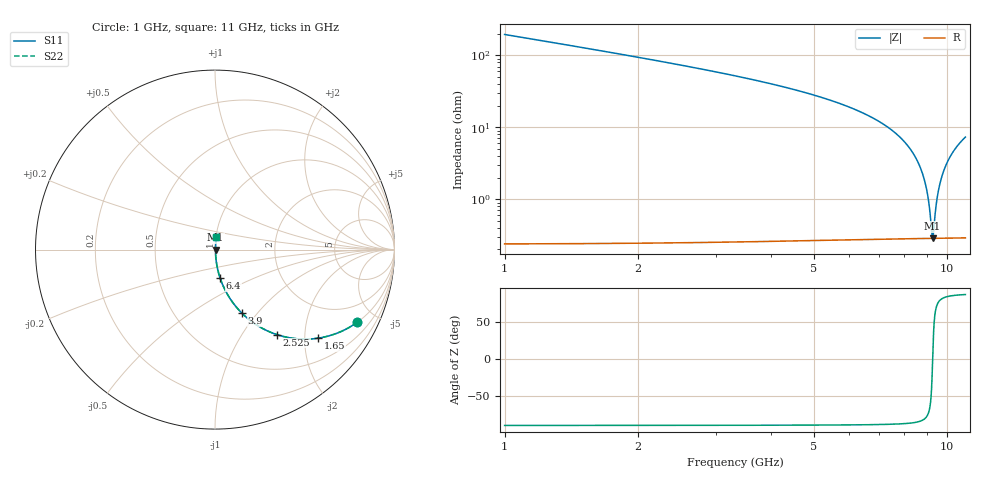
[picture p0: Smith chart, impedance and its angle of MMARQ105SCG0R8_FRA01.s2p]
! MMARQ105SCG0R8_FRA01  S-PARAMETER MODEL  ( General Type )
! Model Generated by TAIYO YUDEN Corporation (http://www.ty-top.com)
! Version 1.0
! TAIYO YUDEN Control No. 200326
! Copyright(c) 2020 TAIYO YUDEN CO.,LTD. All Rights Reserved.
! Product Description (link to TY-COMPAS)
! https://ds.yuden.co.jp/TYCOMPAS/or/detail?pn=MMARQ105SCG0R8BFRA01&u=M
! Products Name : Multilayer Ceramic Capacitors
! Characteristics :
!  Capacitance : 0.8 pF , Rated Voltage : 250V , TCC : CG / C0G
!  Case Size : 1.0 x 0.5 / 0.039 x 0.02 [mm/inch] , Thickness : 0.5 / 0.02 [mm/inch]
!  (Conditions: Temperature = 25 degC , DC Bias Current/Voltage = 0A / 0V)
! External Node Assignments :
!  1  o---| |---o  2
! GND o---------o GND
! Frequency Range : 1GHz  -  11GHz  [ 401 STEP ]
# MHz S RI R 50
! Freq[MHz].  S11 Real  S11 Imag  S21 Real  S21 Imag  S12 Real  S12 Imag  S22 Real  S22 Imag
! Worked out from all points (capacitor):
!   401 points, 1 GHz to 11 GHz, reference 50 ohm
!   read as one part in series: C = 802 fF near 1.05 GHz
!   lowest |Z| = 286 mohm at 9.275 GHz (marker M1)
!   series resonance near 9.276 GHz, so ESL is about 370 pH
!   S11 on the Smith chart (normalised r, x): 1 GHz: 1.00, -3.92; 1.65 GHz: 1.00, -2.33; 2.525 GHz: 1.00, -1.45; 3.9 GHz: 1.01, -0.84; 6.4 GHz: 1.01, -0.32; 11 GHz: 1.01, +0.15
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1000  0.7934 -0.4043  0.2066 0.4043  0.2066 0.4043  0.7934 -0.4043
1650  0.5754 -0.4932  0.4246 0.4932  0.4246 0.4932  0.5754 -0.4932
2525  0.3466 -0.4742  0.6534 0.4742  0.6534 0.4742  0.3466 -0.4742
2675  0.3168 -0.4634  0.6832 0.4634  0.6832 0.4634  0.3168 -0.4634
3900  0.1507 -0.3547  0.8493 0.3547  0.8493 0.3547  0.1507 -0.3547
4350  0.1141 -0.3143  0.8859 0.3143  0.8859 0.3143  0.1141 -0.3143
6000  0.0381 -0.1844  0.9619 0.1844  0.9619 0.1844  0.0381 -0.1844
6400  0.0282 -0.1573  0.9718 0.1573  0.9718 0.1573  0.0282 -0.1573
7675  0.00933 -0.0805  0.9907 0.0805  0.9907 0.0805  0.00933 -0.0805
8325  0.00494 -0.046  0.9951 0.046  0.9951 0.046  0.00494 -0.046
8775  0.00339 -0.0236  0.9966 0.0236  0.9966 0.0236  0.00339 -0.0236
9025  0.00298 -0.0117  0.997 0.0117  0.997 0.0117  0.00298 -0.0117
9125  0.00289 -0.00698  0.9971 0.00698  0.9971 0.00698  0.00289 -0.00698
9225  0.00285 -0.00235  0.9971 0.00235  0.9971 0.00235  0.00285 -0.00235
9275  0.00285 -5.25e-05  0.9972 5.25e-05  0.9972 5.25e-05  0.00285 -5.25e-05
9300  0.00285 0.00109  0.9972 -0.00109  0.9972 -0.00109  0.00285 0.00109
9350  0.00286 0.00337  0.9971 -0.00337  0.9971 -0.00337  0.00286 0.00337
9450  0.00291 0.00789  0.9971 -0.00789  0.9971 -0.00789  0.00291 0.00789
9550  0.00301 0.0124  0.997 -0.0124  0.997 -0.0124  0.00301 0.0124
9850  0.00352 0.0255  0.9965 -0.0255  0.9965 -0.0255  0.00352 0.0255
10325  0.00496 0.0455  0.995 -0.0455  0.995 -0.0455  0.00496 0.0455
11000  0.00817 0.0724  0.9918 -0.0724  0.9918 -0.0724  0.00817 0.0724
